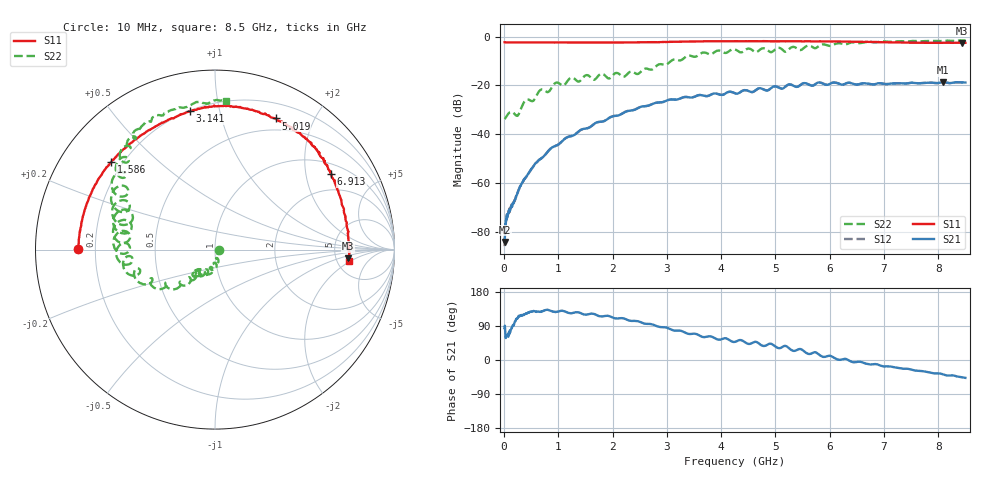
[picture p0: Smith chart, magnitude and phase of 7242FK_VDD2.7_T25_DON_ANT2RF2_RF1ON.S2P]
!Agilent Technologies,E5071C,MY46417908,A.11.23
!Date: Wed Dec 09 15:38:50 2020
!Data & Calibration Information:
!Freq	S11:SOLT2(ON)	S21:SOLT2(ON)	S12:SOLT2(ON)	S22:SOLT2(ON)
!PortZ  Port1:50+j0  Port2:50+j0
!Above PortZ is port z conversion or system Z0 setting when saving the data.
!When reading, reference impedance value at option line is always used.
# Hz S dB R 50
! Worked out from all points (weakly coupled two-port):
!   1601 points, 10 MHz to 8.5 GHz, reference 50 ohm
!   highest |S21| = -18.67 dB at 8.091 GHz (marker M1); lowest = -84.2 dB at 10 MHz (marker M2)
!   lowest |S11| = -2.6 dB at 8.442 GHz (marker M3), VSWR 6.81, Z = 325 - j71.1 ohm
!   |S11| at or under -10 dB: nowhere
!   |S22| runs from -33.8 to -1.6 dB; largest |S21 - S12| = 0.0019
!   S11 on the Smith chart (normalised r, x): 10 MHz: 0.13, +0.00; 1.586 GHz: 0.16, +0.36; 3.141 GHz: 0.20, +0.81; 5.019 GHz: 0.36, +1.50; 6.913 GHz: 1.33, +2.79; 8.5 GHz: 6.34, -1.86
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1e7  -2.34 179.7  -84.20 84.2  -85.95 94.6  -33.79 -0.8
9.49e7  -2.38 177.4  -72.02 67.6  -71.41 73.9  -31.23 -31.5
2.965375e8  -2.39 172.0  -61.39 116.2  -61.44 116.5  -30.45 -50.7
3.973562e8  -2.40 169.3  -57.83 122.4  -57.74 122.3  -26.10 -69.5
5.459312e8  -2.40 165.6  -52.96 129.6  -52.99 129.0  -26.19 -75.8
6.67975e8  -2.40 162.5  -50.18 127.0  -50.24 127.5  -21.89 -82.4
8.1655e8  -2.41 158.7  -46.88 131.8  -46.80 132.1  -22.69 -89.7
9.545125e8  -2.40 155.4  -44.73 126.7  -44.75 126.8  -18.93 -94.6
1.426769e9  -2.41 143.9  -38.12 122.6  -38.12 122.7  -17.56 -107.0
1.585956e9  -2.42 139.8  -37.08 121.8  -37.08 121.8  -16.53 -125.9
2.206788e9  -2.39 123.2  -31.16 109.6  -31.16 109.6  -16.50 -127.5
2.843538e9  -2.28 107.0  -27.03 88.0  -27.04 88.0  -11.47 -131.3
3.140688e9  -2.11 100.4  -25.82 77.5  -25.84 77.5  -9.38 -142.6
4.255e9  -1.86 80.0  -23.26 47.8  -23.26 47.8  -5.26 179.5
4.912975e9  -1.93 66.9  -21.23 43.0  -21.23 43.0  -6.37 165.0
5.0191e9  -1.88 65.2  -20.51 33.4  -20.49 33.4  -4.81 167.4
5.671769e9  -1.96 52.3  -20.13 17.7  -20.07 17.5  -4.11 145.1
6.913431e9  -2.24 33.1  -19.10 -13.6  -19.14 -13.5  -2.13 125.9
7.088538e9  -2.32 29.2  -19.37 -16.7  -19.44 -16.8  -2.12 121.5
8.091419e9  -2.54 3.6  -18.67 -38.1  -18.73 -38.0  -1.77 100.0
8.441631e9  -2.57 -3.8  -18.76 -45.7  -18.85 -45.8  -1.61 87.9
8.5e9  -2.54 -5.0  -18.84 -47.1  -18.95 -46.9  -1.60 85.9
